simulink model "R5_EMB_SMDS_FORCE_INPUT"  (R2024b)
settings: Solver=FixedStepDiscrete  StartTime=0.0  StopTime=S  FixedStep=T  RelTol=1e-3  EnableMultiTasking=on
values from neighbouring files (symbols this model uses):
  Kt = Kt*motor_eff    (= 0.0273)    [R5_EMB_SMDS_FORCE_INPUT_script.m]
  r = 0.01    [R5_EMB_SMDS_FORCE_INPUT_script.m]
  T = 0.002    [R5_EMB_SMDS_FORCE_INPUT_script.m]
undefined symbols (not defined in the file or in its folder): Serial_Port, Standard_Devices
libraries: easyio x6, simulink x3

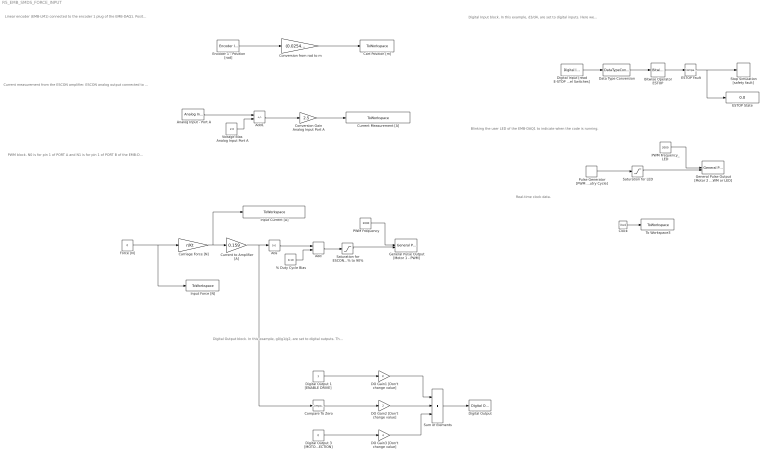
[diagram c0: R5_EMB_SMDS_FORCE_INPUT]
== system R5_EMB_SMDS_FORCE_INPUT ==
  note: Current measurement from the ESCON amplifier. ESCON analog output connected to pin 5 of PORT A (analog in).
  note: Linear encoder (EMB-LM1) connected to the encoder 1 plug of the EMB-DAQ1. Position reading with units in meters [m].
  note: Digital Output block. In this example, g0/g1/g2, are set to digital outputs. The gains are related to each output pin (gain =1 for g0, gain=2 for g1, gain=4 for g2) and the sum is fed to G0 block. Here we used constants for g0 and g2. For g1, we take the signal of the input force to determine the direction of the motor.
  note: Digital Input block. In this example, d3/d4, are set to digital inputs. Here we used these digital inputs for a safety system. The E-STOP is d3 and the End-of-Travel Switch is d4 (EoTS). To isolate these states from the digital inputs, a Bitwise AND operation is performed. Since the Simulink Bitwise Operator accepts only integer data types, the signal is first converted to an unsigned 8-bit integer (uint8). We stop the simulation if the E-STOPis pressed. No EoTS in this model.
  note: PWM block. N0 is for pin 1 of PORT A and N1 is for pin 1 of PORT B of the EMB-DAQ1. We set the PWM mode to frequency and duty. The ESCON frequency range is from 10Hz to 5KHz and the duty is from 0.1 and 0.9%.
  note: Real-time clock data.
  note: Blinking the user LED of the EMB-DAQ1 to indicate when the code is running.
  % Duty Cycle Bias : Constant  Value=0.10
  Abs : Abs
  Add : Sum
  Add1 : Sum  Inputs=+-
  Analog Input - Port A : easyio/Analog Input  SampleTime=T  MaxMissedTicks=10  ShowMissedTicks=0  YieldWhenWaiting=0  DrvName=Standard_Devices/Serial_Port  DrvAddress=6  DrvOptions=[460800 8 0 0 0 0 0 0]  PacketSize=8  DataTypes='double'  ShowReady=0  ShowError=0  PacketID=1  ByteOrder=1  ShowTimestamp=0  CfgPrm=A6  PrmCfg=unipolar  ResVar=0  VarRes=0
  Bitwise Operator ESTOP : simulink/Logic and Bit Operations/Bitwise Operator  logicop=AND  UseBitMask=on  BitMask=8  BitMaskRealWorld=Real World Value
  Carriage Force [N] : Gain  Gain=r/Kt
  Cart Position [m] : ToWorkspace  VariableName=cart_position  SampleTime=-1
  Clock : Clock
  Compare To Zero : simulink/Logic and Bit Operations/Compare To Zero  relop=>=  OutDataTypeStr=boolean
  Conversion Gain Analog Input Port A : Gain  Gain=2.5
  Conversion from rad to m : Gain  Gain=(0.0254)/(2*pi)
  Current Measurement [A] : ToWorkspace  VariableName=i_measure  SampleTime=-1
  Current to Amplifier [A] : Gain  Gain=0.159
  DO Gain1 [Don't change value] : Gain
  DO Gain2 [Don't change value] : Gain  Gain=2
  DO Gain3 [Don't change value] : Gain  Gain=4
  Data Type Conversion : DataTypeConversion  OutDataTypeStr=uint8  RndMeth=Nearest
  Digital Input [read E-STOP and End of Travel Switches] : easyio/Digital Input  SampleTime=T  MaxMissedTicks=10  ShowMissedTicks=0  YieldWhenWaiting=0  DrvName=Standard_Devices/Serial_Port  DrvAddress=6  DrvOptions=[460800 8 0 0 0 0 0 0]  PacketSize=8  DataTypes='double'  ShowReady=0  ShowError=0  PacketID=1  ByteOrder=1  ShowTimestamp=0  CfgPrm=D0  PrmCfg=18  ResVar=0  VarRes=0  d7=off  d6=off  d5=off  d4=on  d3=on  d2=off  d1=off  d0=off
  Digital Output : easyio/Digital Output  SampleTime=T  MaxMissedTicks=10  ShowMissedTicks=0  YieldWhenWaiting=0  DrvName=Standard_Devices/Serial_Port  DrvAddress=6  DrvOptions=[460800 8 0 0 0 0 0 0]  PacketSize=8  DataTypes='double'  ShowReady=0  ShowError=0  PacketID=1  ByteOrder=1  InitialValue=0  FinalValue=0  CfgPrm=G0  PrmCfg=F8  ResVar=0  VarRes=0  d7=off  d6=off  d5=off  d4=off  d3=off  d2=on  d1=on  d0=on
  Digital Output 1 [ENABLE DRIVE] : Constant
  Digital Output 3 [MOTOR 2 DIRECTION] : Constant  Value=0
  ESTOP Fault : simulink/Logic and Bit Operations/Compare To Constant  relop=~=  const=8  OutDataTypeStr=boolean
  ESTOP State : Display
  Encoder 1 - Position [rad] : easyio/Encoder Input  SampleTime=T  MaxMissedTicks=10  ShowMissedTicks=0  YieldWhenWaiting=0  DrvName=Standard_Devices/Serial_Port  DrvAddress=6  DrvOptions=[460800 8 0 0 0 0 0 0]  PacketSize=8  DataTypes='double'  ShowReady=0  ShowError=0  PacketID=1  ByteOrder=1  ShowTimestamp=0  CfgPrm=E0  PrmCfg=position  ResVar=0  VarRes=2000
  Force [N] : Constant  Value=0
  General Pulse Output [Motor 1 - PWM] : easyio/General Pulse Output  SampleTime=T  MaxMissedTicks=10  ShowMissedTicks=0  YieldWhenWaiting=0  DrvName=Standard_Devices/Serial_Port  DrvAddress=6  DrvOptions=[460800 8 0 0 0 0 0 0]  PacketSize=16  DataTypes={'double','double'}  ShowReady=0  ShowError=0  PacketID=1  ByteOrder=1  InitialValue=[0 0]  FinalValue=[0 0]  CfgPrm=N0  PrmCfg=frequency and duty  ResVar=449.8360 Hz - 115156.25 Hz  VarRes=64
  General Pulse Output [Motor 2 - PWM or LED] : easyio/General Pulse Output  SampleTime=T  MaxMissedTicks=10  ShowMissedTicks=0  YieldWhenWaiting=0  DrvName=Standard_Devices/Serial_Port  DrvAddress=6  DrvOptions=[460800 8 0 0 0 0 0 0]  PacketSize=16  DataTypes={'double','double'}  ShowReady=0  ShowError=0  PacketID=1  ByteOrder=1  InitialValue=[0 0]  FinalValue=[0 0]  CfgPrm=N1  PrmCfg=frequency and duty  ResVar=449.8360 Hz - 115156.25 Hz  VarRes=64
  Input Current [A] : ToWorkspace  VariableName=i_input  SampleTime=-1
  Input Force [N] : ToWorkspace  VariableName=f_input  SampleTime=-1
  PWM Frequency : Constant  Value=2000
  PWM Frequency_LED : Constant  Value=2000
  Pulse Generator [PWM % Dutry Cycle] : DiscretePulseGenerator  PulseType=Time based  Period=0.4  PulseWidth=50
  Saturation for ESCON 10% to 90% : Saturate  UpperLimit=0.9  LowerLimit=0.1
  Saturation for LED : Saturate  UpperLimit=1  LowerLimit=0
  Stop Simulation [safety fault] : Stop
  Sum of Elements : Sum  Inputs=+++
  To Workspace3 : ToWorkspace  VariableName=rt_time  SampleTime=-1
  Voltage Bias Analog Input Port A : Constant  Value=2.0
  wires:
  Encoder 1 - Position [rad]/1 -> Conversion from rad to m/1
  PWM Frequency/1 -> General Pulse Output [Motor 1 - PWM]/1
  Digital Output 1 [ENABLE DRIVE]/1 -> DO Gain1 [Don't change value]/1
  Sum of Elements/1 -> Digital Output/1
  DO Gain2 [Don't change value]/1 -> Sum of Elements/2
  DO Gain1 [Don't change value]/1 -> Sum of Elements/1
  Saturation for LED/1 -> General Pulse Output [Motor 2 - PWM or LED]/2
  Pulse Generator [PWM % Dutry Cycle]/1 -> Saturation for LED/1
  Digital Output 3 [MOTOR 2 DIRECTION]/1 -> DO Gain3 [Don't change value]/1
  DO Gain3 [Don't change value]/1 -> Sum of Elements/3
  Voltage Bias Analog Input Port A/1 -> Add1/2
  Analog Input - Port A/1 -> Add1/1
  Conversion from rad to m/1 -> Cart Position [m]/1
  Clock/1 -> To Workspace3/1
  Abs/1 -> Add/1
  Saturation for ESCON 10% to 90%/1 -> General Pulse Output [Motor 1 - PWM]/2
  Current to Amplifier [A]/1 -> Compare To Zero/1, Abs/1
  % Duty Cycle Bias/1 -> Add/2
  Add/1 -> Saturation for ESCON 10% to 90%/1
  Compare To Zero/1 -> DO Gain2 [Don't change value]/1
  PWM Frequency_LED/1 -> General Pulse Output [Motor 2 - PWM or LED]/1
  Force [N]/1 -> Carriage Force [N]/1, Input Force [N]/1
  Carriage Force [N]/1 -> Input Current [A]/1, Current to Amplifier [A]/1
  Conversion Gain Analog Input Port A/1 -> Current Measurement [A]/1
  Bitwise Operator ESTOP/1 -> ESTOP Fault/1
  ESTOP Fault/1 -> ESTOP State/1, Stop Simulation [safety fault]/1
  Data Type Conversion/1 -> Bitwise Operator ESTOP/1
  Digital Input [read E-STOP and End of Travel Switches]/1 -> Data Type Conversion/1
  Add1/1 -> Conversion Gain Analog Input Port A/1
